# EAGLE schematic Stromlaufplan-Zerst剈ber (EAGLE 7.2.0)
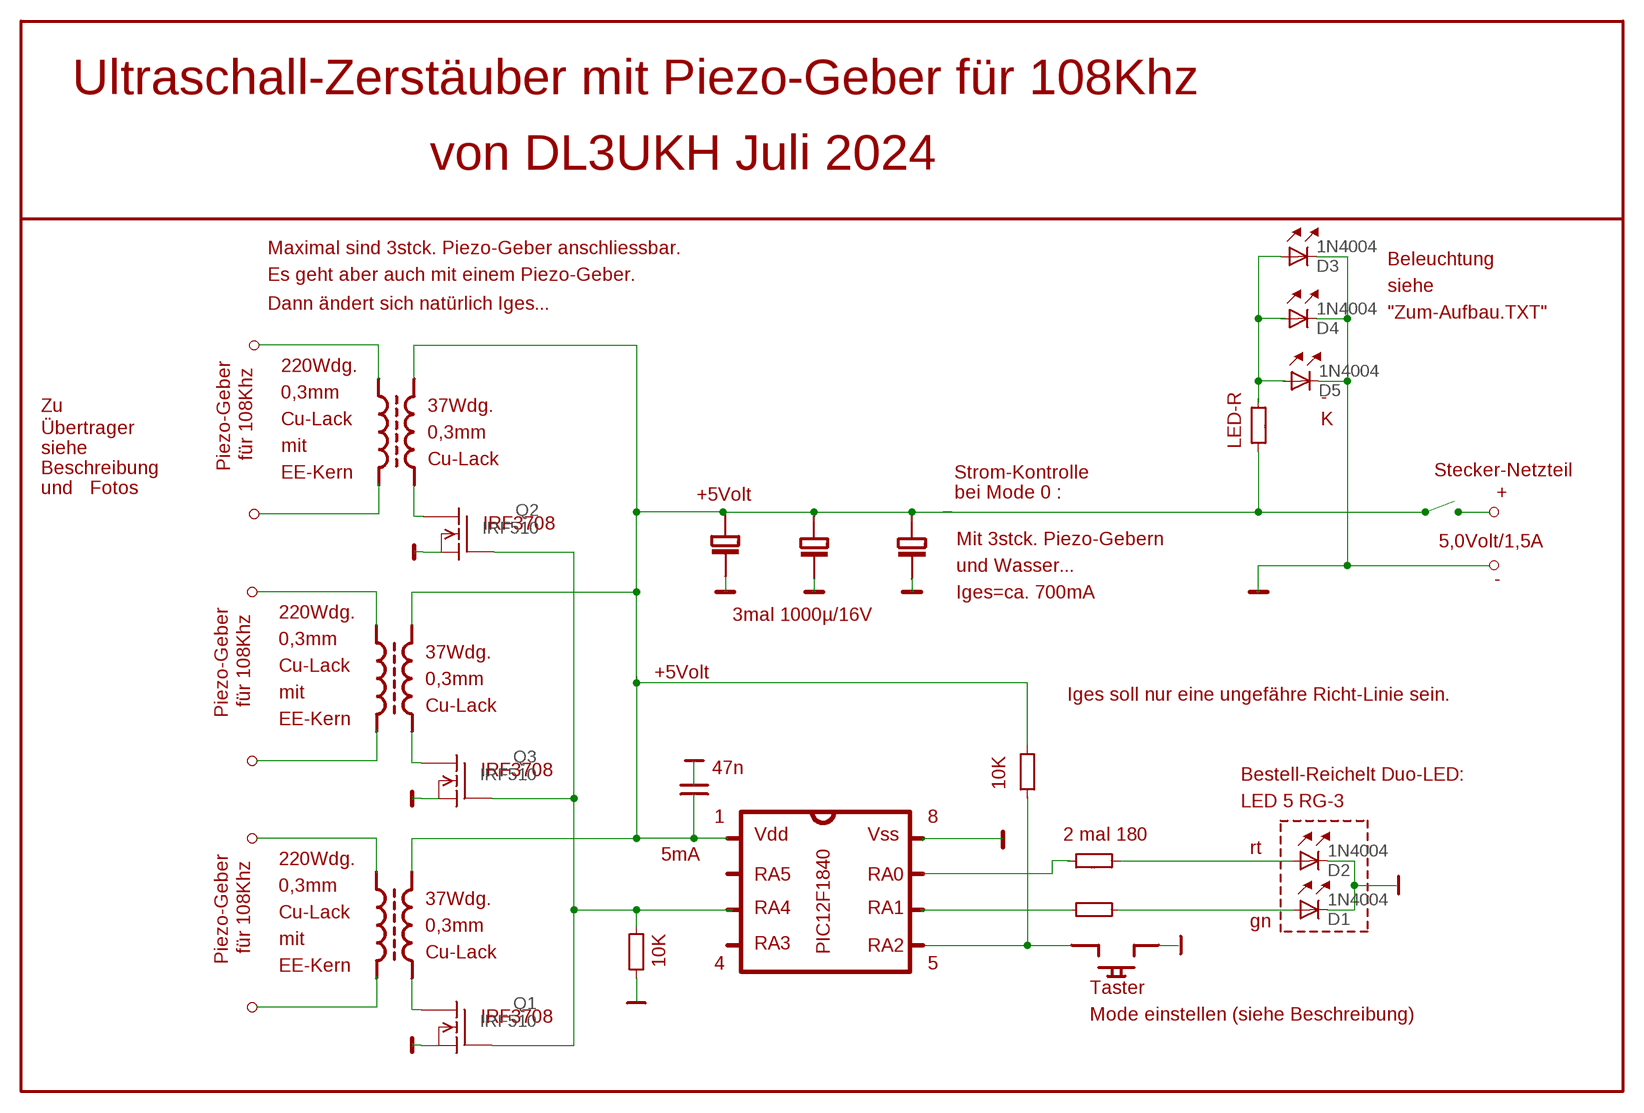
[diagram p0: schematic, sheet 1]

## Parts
D1  1N4004  [DO41-10]
D2  1N4004  [DO41-10]
D3  1N4004  [DO41-10]
D4  1N4004  [DO41-10]
D5  1N4004  [DO41-10]
Q1  IRF510  [TO220]
Q2  IRF510  [TO220]
Q3  IRF510  [TO220]

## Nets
N$5: D1.A D2.A
N$8: D1.C D2.C
N$10: Q1.1(G) Q2.1(G) Q3.1(G)
N$11: Q1.2(D)
N$12: Q1.3(S)
N$19: D3.A D4.A D5.A
N$21: Q3.2(D)
N$23: Q3.3(S)
N$26: Q2.2(D)
N$27: Q2.3(S)
N$49: D3.C D4.C D5.C

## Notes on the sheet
- Ultraschall-Zerstäuber mit Piezo-Geber für 108Khz
- von DL3UKH Juli 2024
- Maximal sind 3stck. Piezo-Geber anschliessbar.
- Beleuchtung
- Es geht aber auch mit einem Piezo-Geber.
- siehe
- Dann ändert sich natürlich Iges...
- "Zum-Aufbau.TXT"
- Piezo-Geber
- für 108Khz | 220Wdg.
- LED-R
- 0,3mm | -
- Zu | 37Wdg.
- Cu-Lack | K
- Übertrager | 0,3mm
- siehe | mit
- Cu-Lack
- Beschreibung | EE-Kern | Strom-Kontrolle | Stecker-Netzteil
- und | Fotos | bei Mode 0 : | +
- +5Volt
- IRF3708
- Mit 3stck. Piezo-Gebern | 5,0Volt/1,5A
- und Wasser...
- -
- Iges=ca. 700mA
- Piezo-Geber | 3mal 1000µ/16V
- für 108Khz | 220Wdg.
- 0,3mm
- 37Wdg.
- Cu-Lack
- +5Volt
- 0,3mm
- mit | Iges soll nur eine ungefähre Richt-Linie sein.
- Cu-Lack
- EE-Kern
- IRF3708 | 47n
- Bestell-Reichelt Duo-LED:
- 10K
- LED 5 RG-3
- 1 | 8
- Vdd | Vss | 2 mal 180
- Piezo-Geber | rt
- für 108Khz | 220Wdg. | 5mA
- RA5 | RA0
- 0,3mm
- 37Wdg.
- Cu-Lack | RA4 | RA1
- 0,3mm | gn
- mit | RA3
- PIC12F1840 | RA2
- Cu-Lack
- EE-Kern | 10K | 4 | 5
- Taster
- IRF3708 | Mode einstellen (siehe Beschreibung)

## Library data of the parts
D1-D5 = diode:1N4004: DIODE
Q1-Q3 = transistor-fet:IRF510: N-Channel Enhancement MOSFET (HEXFET); 100V; 5,6A; 0,54Ohm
